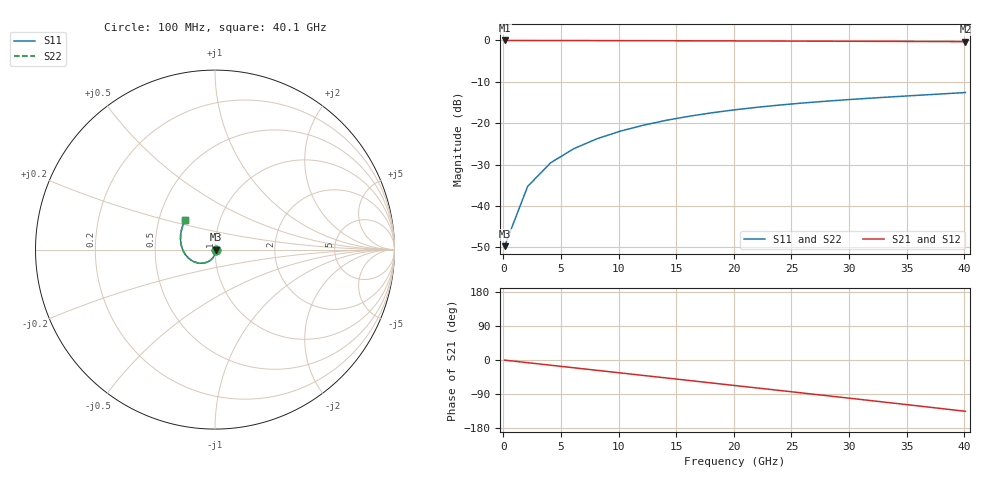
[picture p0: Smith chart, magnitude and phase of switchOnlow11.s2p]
# GHZ S RI R 50
!Output file by Shape3_31
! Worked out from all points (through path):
!   21 points, 100 MHz to 40.1 GHz, reference 50 ohm
!   highest |S21| = -0.03 dB at 100 MHz (marker M1); lowest = -0.3 dB at 40.1 GHz (marker M2)
!   group delay of S21, straight-line fit = 9.35 ps
!   lowest |S11| = -49.7 dB at 100 MHz (marker M3), VSWR 1.01, Z = 50.3 - j0.0614 ohm
!   |S11| at or under -10 dB: start of sweep to end of sweep
!   |S22| runs from -49.7 to -12.6 dB; largest |S21 - S12| = 3.3e-14
0.1  0.00321 -0.00061  0.996 -0.00606  0.996 -0.00606  0.00321 -0.00061
2.1  0.00207 -0.0171  0.9874 -0.1225  0.9874 -0.1225  0.00207 -0.0171
4.1  -0.00366 -0.033  0.9657 -0.2369  0.9657 -0.2369  -0.00366 -0.033
6.1  -0.013 -0.0473  0.9307 -0.3478  0.9307 -0.3478  -0.013 -0.0473
8.1  -0.0255 -0.0593  0.8828 -0.4536  0.8828 -0.4536  -0.0255 -0.0593
10.1  -0.0407 -0.0684  0.8229 -0.5528  0.8229 -0.5528  -0.0407 -0.0684
12.1  -0.0578 -0.0742  0.7517 -0.6441  0.7517 -0.6441  -0.0578 -0.0742
14.1  -0.0763 -0.0763  0.6705 -0.7263  0.6705 -0.7263  -0.0763 -0.0763
16.1  -0.0953 -0.0745  0.5803 -0.7981  0.5803 -0.7981  -0.0953 -0.0745
18.1  -0.1142 -0.0689  0.4824 -0.8588  0.4824 -0.8588  -0.1142 -0.0689
20.1  -0.1322 -0.0594  0.3783 -0.9076  0.3783 -0.9076  -0.1322 -0.0594
22.1  -0.1487 -0.0464  0.2692 -0.9438  0.2692 -0.9438  -0.1487 -0.0464
24.1  -0.1631 -0.0302  0.1568 -0.967  0.1568 -0.967  -0.1631 -0.0302
26.1  -0.1751 -0.0111  0.0423 -0.9769  0.0423 -0.9769  -0.1751 -0.0111
28.1  -0.1841 0.0103  -0.0725 -0.9733  -0.0725 -0.9733  -0.1841 0.0103
30.1  -0.1899 0.0338  -0.1864 -0.9562  -0.1864 -0.9562  -0.1899 0.0338
32.1  -0.1923 0.0587  -0.2976 -0.9256  -0.2976 -0.9256  -0.1923 0.0587
34.1  -0.1912 0.0847  -0.4046 -0.8819  -0.4046 -0.8819  -0.1912 0.0847
36.1  -0.1864 0.1114  -0.506 -0.8254  -0.506 -0.8254  -0.1865 0.1114
38.1  -0.178 0.1384  -0.6001 -0.7568  -0.6001 -0.7568  -0.178 0.1384
40.1  -0.1658 0.1653  -0.6854 -0.6768  -0.6854 -0.6768  -0.1658 0.1653
